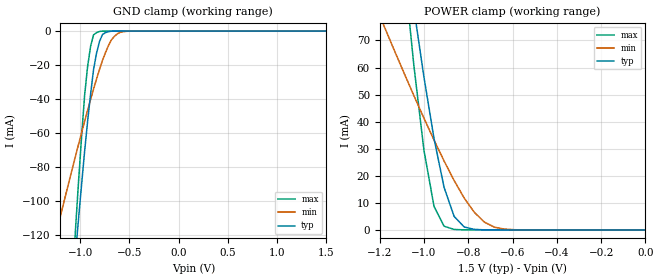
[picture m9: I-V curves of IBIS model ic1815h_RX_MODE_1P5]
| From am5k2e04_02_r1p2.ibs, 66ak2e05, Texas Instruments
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|   Model Cell ic1815h_RX_MODE_1P5
|RX_MODE_1P5
[Model]   ic1815h_RX_MODE_1P5
Model_type   Input
Polarity   Non-Inverting
Vinl =  0.525
Vinh =  0.975
C_comp   0.756654p   0.691399p   0.775102p
[Model Spec]
Vinl   0.525   0.4725   0.5775
Vinh   0.975   0.8775   1.0725
[Temperature Range]   25   125   -40
[Voltage Range]   1.5   1.35   1.65
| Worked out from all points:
|   GND clamp passes 1 mA (typ) near -0.74 V on its own axis
|   POWER clamp passes 1 mA (typ) near -0.81 V on its own axis
[POWER_clamp]
|   voltage   I(typ)   I(min)   I(max)
-1.5V     376.6mA    139.1mA    483.3mA
-1.182V   165.7mA    75.67mA    178.1mA
-1.167V   156.1mA    72.74mA    164.3mA
-1.061V   90.9mA     52.5mA     73.03mA
-1.03V    73.44mA    46.87mA    50.36mA
-1V       56.52mA    41.31mA    29.5mA
-954.5mV  33.82mA    33.23mA    8.736mA
-909.1mV  15.75mA    25.49mA    1.394mA
-863.6mV  5mA        18.27mA    187.8uA
-818.2mV  1.11mA     11.8mA     40.91uA
-681.8mV  15.4uA     1.028mA    13.58uA
0V        38.51pA    138.6pA    41.75pA
[GND_clamp]
|   voltage   I(typ)   I(min)   I(max)
-1.5V     -462.9mA   -179.7mA   -593.8mA
-1.227V   -259.3mA   -114.9mA   -299.5mA
-1.045V   -129.9mA   -73.08mA   -115mA
-1.015V   -109.6mA   -66.33mA   -87.45mA
-954.5mV  -70.65mA   -53.01mA   -37.72mA
-924.2mV  -53.14mA   -46.56mA   -20.82mA
-863.6mV  -22.55mA   -34.01mA   -2.188mA
-833.3mV  -12.92mA   -28.14mA   -922.9uA
-772.7mV  -1.992mA   -17.16mA   -44.91uA
-681.8mV  -79.59uA   -5.101mA   -8.29uA
-590.9mV  -4.252uA   -672.1uA   -3.267uA
1.5V      38.51pA    2.566nA    35.42pA
